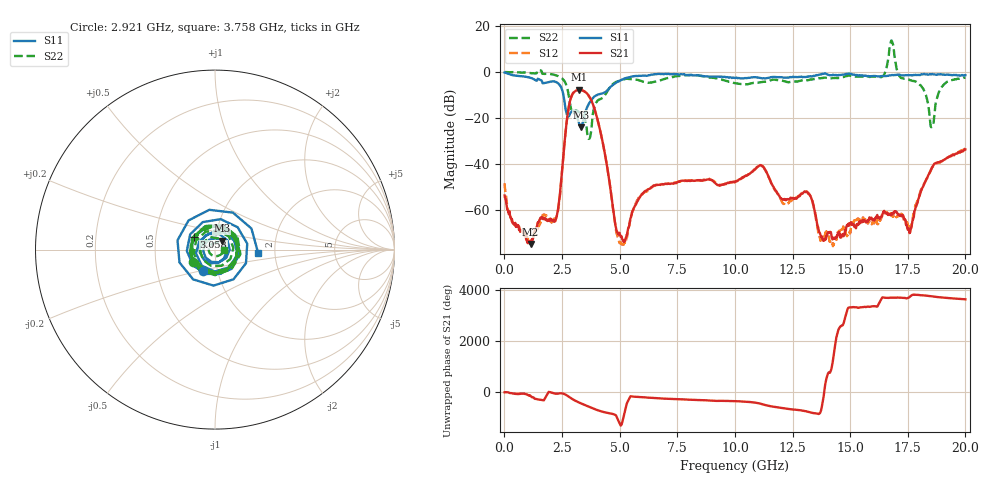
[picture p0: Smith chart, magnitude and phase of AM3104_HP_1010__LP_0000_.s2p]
!Created with skrf (http://scikit-rf.org).
# Hz S RI R 50.0
!freq ReS11 ImS11 ReS21 ImS21 ReS12 ImS12 ReS22 ImS22
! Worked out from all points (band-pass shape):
!   1601 points, 10 MHz to 20 GHz, reference 50 ohm
!   highest |S21| = -7.76 dB at 3.258 GHz (marker M1); lowest = -74.7 dB at 1.134 GHz (marker M2)
!   |S21| within 3 dB of the highest: 2.904 GHz to 3.69 GHz (786.3 MHz wide, 23.9 % of centre)
!   lowest |S11| = -24.0 dB at 3.333 GHz (marker M3), VSWR 1.13, Z = 53.7 + j5.4 ohm
!   |S11| at or under -10 dB: 2.56 GHz to 4.026 GHz (1.466 GHz wide, 44.5 % of centre)
!   |S22| runs from -29.1 to 13.7 dB; largest |S21 - S12| = 0.02
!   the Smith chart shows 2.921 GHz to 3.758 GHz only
!   S11 on the Smith chart (normalised r, x): 2.921 GHz: 0.85, -0.21; 3.058 GHz: 0.78, +0.11; 3.758 GHz: 1.63, -0.06
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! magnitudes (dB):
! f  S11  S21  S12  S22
! 10 MHz  -0.2  -53.7  -48.4  0.0
! 1.134 GHz  -2.5  -74.7  -73.6  -0.5
! 2.246 GHz  -4.4  -63.7  -63.2  -1.5
! 2.921 GHz  -17.2  -10.3  -10.4  -16.9
! 3.058 GHz  -17.2  -8.4  -8.4  -17.0
! 3.258 GHz  -23.0  -7.8  -7.9  -17.6
! 3.333 GHz  -24.0  -7.9  -8.0  -17.8
! 3.346 GHz  -24.0  -7.9  -8.0  -17.9
! 3.758 GHz  -12.4  -12.0  -12.1  -26.2
! 5.045 GHz  -3.6  -71.7  -73.9  -3.7
! 6.682 GHz  -0.9  -49.1  -49.0  -3.9
! 10.01 GHz  -2.6  -47.9  -47.8  -4.9
! 11.14 GHz  -2.7  -40.6  -40.7  -4.5
! 12.12 GHz  -2.4  -55.5  -57.3  -4.0
! 13.34 GHz  -1.9  -55.6  -55.7  -3.3
! 13.75 GHz  -1.0  -71.9  -72.8  -2.6
! 14.2 GHz  -1.4  -72.0  -74.1  -2.8
! 16.68 GHz  -1.5  -62.1  -62.1  7.2
! 17.59 GHz  -1.4  -69.7  -66.9  -3.5
! 18.54 GHz  -0.9  -41.7  -42.0  -24.0
! 19 GHz  -1.2  -38.7  -38.7  -6.2
! 20 GHz  -1.4  -33.6  -33.4  -2.5
